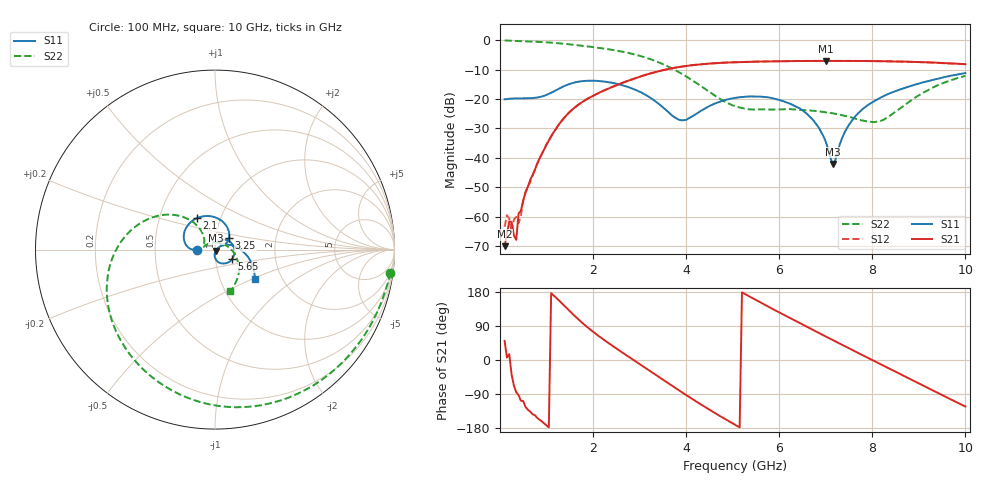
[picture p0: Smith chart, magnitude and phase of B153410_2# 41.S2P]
!  2-Port S-parameters saved by WinCal
! VAR MeasName=S-Parameters (CALIBRATED_DATA) read from VNA (N5245A)
! VAR MeasDate=2016-12-23 10:01:29
! VAR NAME=B153410_2# 41
! VAR FILENAME=B153410_2# 41.S2P
! VAR DATE=2016-12-23 10:01:29
! VAR PHYS_PORTS=1,2
# Hz S DB R 50
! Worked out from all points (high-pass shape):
!   199 points, 100 MHz to 10 GHz, reference 50 ohm
!   highest |S21| = -7.05 dB at 7 GHz (marker M1); lowest = -70.0 dB at 100 MHz (marker M2)
!   |S21| within 3 dB of the highest: 3.551 GHz to end of sweep
!   lowest |S11| = -42.1 dB at 7.15 GHz (marker M3), VSWR 1.02, Z = 50.6 - j0.521 ohm
!   |S11| at or under -10 dB: start of sweep to end of sweep
!   |S22| runs from -27.9 to -0.1 dB; largest |S21 - S12| = 0.0039
!   S11 on the Smith chart (normalised r, x): 100 MHz: 0.82, -0.00; 2.1 GHz: 0.77, +0.28; 3.25 GHz: 1.16, +0.15; 5.65 GHz: 1.20, -0.13; 10 GHz: 1.46, -0.52
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1e8  -20.12 -178.5  -70.02 50.5  -63.46 66.4  -0.13 -7.5
1.5e8  -20.06 -178.9  -65.79 6.4  -59.52 -18.1  -0.17 -11.0
2e8  -19.93 -179.6  -61.63 15.6  -60.71 34.8  -0.22 -14.3
2.5e8  -19.88 179.9  -61.80 -38.4  -65.52 -57.8  -0.25 -17.7
3.5e8  -19.81 178.7  -67.89 -85.0  -60.08 -62.7  -0.31 -24.3
4e8  -19.84 178.1  -58.94 -92.7  -62.23 -105.9  -0.34 -27.6
6e8  -19.77 177.3  -49.85 -131.2  -49.67 -132.9  -0.46 -40.8
1e9  -18.61 -180.0  -35.55 -172.9  -35.43 -172.4  -0.76 -66.8
1.75e9  -13.97 145.6  -21.25 100.1  -21.23 100.2  -1.90 -112.6
2.1e9  -13.88 120.2  -18.10 65.2  -18.13 65.4  -2.59 -132.2
3.25e9  -19.81 40.2  -11.25 -31.2  -11.25 -31.1  -6.59 165.0
3.4e9  -21.51 32.8  -10.63 -43.5  -10.61 -43.5  -7.51 157.4
3.95e9  -27.21 46.2  -8.91 -88.4  -8.91 -88.4  -11.86 134.4
5.05e9  -19.66 11.3  -7.53 -171.0  -7.54 -170.9  -22.44 142.3
5.65e9  -19.28 -29.8  -7.30 148.2  -7.28 148.3  -23.51 162.7
6.7e9  -26.66 -89.5  -7.06 80.8  -7.07 80.9  -23.98 163.9
7e9  -34.55 -91.9  -7.05 61.9  -7.06 62.1  -24.57 159.0
7.15e9  -42.09 -40.9  -7.08 52.6  -7.05 52.7  -24.87 154.5
7.6e9  -26.53 28.6  -7.07 24.6  -7.09 24.7  -26.53 133.9
8.35e9  -18.26 6.2  -7.23 -21.8  -7.22 -21.5  -25.98 44.7
9.2e9  -13.93 -16.1  -7.56 -74.0  -7.58 -74.0  -16.98 -26.8
1e10  -11.19 -36.7  -8.20 -122.8  -8.20 -122.3  -12.18 -69.9
